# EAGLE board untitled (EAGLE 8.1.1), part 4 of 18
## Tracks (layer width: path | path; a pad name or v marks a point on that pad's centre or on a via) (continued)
S$3328 (continued)
  Bottom 0: 233.07,164.65 233.19,164.95
S$3329
  Bottom 0: 233.19,164.95 233.24,165.27
S$3330
  Bottom 0: 233.24,165.27 233.19,165.59
S$3331
  Bottom 0: 233.19,165.59 233.07,165.89
S$3332
  Bottom 0: 233.07,165.89 232.86,166.14
S$3333
  Bottom 0: 232.86,166.14 232.6,166.33
S$3334
  Bottom 0: 232.6,166.33 232.29,166.44
S$3335
  Bottom 0: 232.29,166.44 232.18,166.44
S$3336
  Bottom 0: 232.18,166.44 232.18,167.7
S$3337
  Bottom 0: 232.18,167.7 232.41,167.45
S$3338
  Bottom 0: 232.41,167.45 232.71,167.26
S$3339
  Bottom 0: 232.71,167.26 233.03,167.16
S$3340
  Bottom 0: 233.03,167.16 233.38,167.14
S$3341
  Bottom 0: 233.38,167.14 233.73,167.2
S$3342
  Bottom 0: 233.73,167.2 234.05,167.35
S$3343
  Bottom 0: 234.05,167.35 234.31,167.57
S$3344
  Bottom 0: 234.31,167.57 234.52,167.86
S$3345
  Bottom 0: 234.52,167.86 234.65,168.18
S$3346
  Bottom 0: 234.65,168.18 234.7,168.53
S$3347
  Bottom 0: 234.7,168.53 234.65,168.87
S$3348
  Bottom 0: 234.65,168.87 234.52,169.2
S$3349
  Bottom 0: 234.52,169.2 234.31,169.48
S$3350
  Bottom 0: 234.31,169.48 234.05,169.71
S$3351
  Bottom 0: 234.05,169.71 233.73,169.86
S$3352
  Bottom 0: 233.73,169.86 233.38,169.92
S$3353
  Bottom 0: 233.38,169.92 233.03,169.9
S$3354
  Bottom 0: 233.03,169.9 232.71,169.79
S$3355
  Bottom 0: 232.71,169.79 232.41,169.61
S$3356
  Bottom 0: 232.41,169.61 232.18,169.36
S$3357
  Bottom 0: 232.18,169.36 232.18,174.4
S$3358
  Bottom 0: 232.18,174.4 234.88,177.1
S$3359
  Bottom 0: 234.88,177.1 234.93,177.17
S$3360
  Bottom 0: 234.93,177.17 234.95,177.2
S$3361
  Bottom 0: 234.95,177.2 234.96,177.24
S$3362
  Bottom 0: 234.96,177.24 235,177.3
S$3363
  Bottom 0: 235,177.3 235,177.36
S$3364
  Bottom 0: 235,177.36 235.01,177.42
S$3365
  Bottom 0: 235.01,177.42 235.01,177.55
S$3366
  Bottom 0: 235.01,177.55 235.46,177.55
S$3367
  Bottom 0: 235.46,177.55 235.53,177.56
S$3368
  Bottom 0: 235.53,177.56 235.6,177.6
S$3369
  Bottom 0: 235.6,177.6 235.66,177.65
S$3370
  Bottom 0: 235.66,177.65 235.7,177.72
S$3371
  Bottom 0: 235.7,177.72 235.71,177.8
S$3372
  Bottom 0: 235.71,177.8 235.71,179.58
S$3373
  Bottom 0: 235.71,179.58 235.7,179.65
S$3374
  Bottom 0: 235.7,179.65 235.66,179.72
S$3375
  Bottom 0: 235.66,179.72 235.6,179.78
S$3376
  Bottom 0: 235.6,179.78 235.53,179.82
S$3377
  Bottom 0: 235.53,179.82 235.46,179.83
S$3378
  Bottom 0: 235.46,179.83 233.68,179.83
S$3379
  Bottom 0: 233.68,179.83 233.6,179.82
S$3380
  Bottom 0: 233.6,179.82 233.53,179.78
S$3381
  Bottom 0: 233.53,179.78 233.48,179.72
S$3382
  Bottom 0: 233.48,179.72 233.44,179.65
S$3383
  Bottom 0: 233.44,179.65 233.43,179.58
S$3384
  Bottom 0: 233.43,179.58 233.43,177.8
S$3385
  Bottom 0: 233.43,177.8 233.44,177.72
S$3386
  Bottom 0: 233.44,177.72 233.48,177.65
S$3387
  Bottom 0: 233.48,177.65 233.53,177.6
S$3388
  Bottom 0: 233.53,177.6 233.6,177.56
S$3389
  Bottom 0: 233.6,177.56 233.68,177.55
S$3390
  Bottom 0: 233.68,177.55 234.07,177.55
S$3391
  Bottom 0: 234.07,177.55 231.42,174.9
S$3392
  Bottom 0: 231.42,174.9 231.38,174.84
S$3393
  Bottom 0: 231.38,174.84 231.34,174.78
S$3394
  Bottom 0: 231.34,174.78 231.31,174.72
S$3395
  Bottom 0: 231.31,174.72 231.29,174.66
S$3396
  Bottom 0: 231.29,174.66 231.29,174.58
S$3397
  Bottom 0: 231.29,174.58 231.29,166.18
S$3398
  Bottom 0: 231.29,166.18 231.12,166.02
S$3399
  Bottom 0: 231.12,166.02 230.95,165.75
S$3400
  Bottom 0: 230.95,165.75 230.87,165.43
S$3401
  Bottom 0: 230.87,165.43 230.87,165.1
S$3402
  Bottom 0: 230.87,165.1 230.95,164.79
S$3403
  Bottom 0: 230.95,164.79 231.12,164.52
S$3404
  Bottom 0: 231.12,164.52 231.36,164.29
S$3405
  Bottom 0: 231.36,164.29 231.65,164.15
S$3406
  Bottom 0: 231.65,164.15 231.97,164.08
S$3407
  Bottom 0: 239.59,164.08 239.92,164.1
S$3408
  Bottom 0: 239.92,164.1 240.22,164.21
S$3409
  Bottom 0: 240.22,164.21 240.49,164.39
S$3410
  Bottom 0: 240.49,164.39 240.69,164.65
S$3411
  Bottom 0: 240.69,164.65 240.82,164.95
S$3412
  Bottom 0: 240.82,164.95 240.87,165.27
S$3413
  Bottom 0: 240.87,165.27 240.82,165.59
S$3414
  Bottom 0: 240.82,165.59 240.69,165.89
S$3415
  Bottom 0: 240.69,165.89 240.49,166.14
S$3416
  Bottom 0: 240.49,166.14 240.22,166.33
S$3417
  Bottom 0: 240.22,166.33 239.92,166.44
S$3418
  Bottom 0: 239.92,166.44 239.59,166.46
S$3419
  Bottom 0: 239.59,166.46 239.27,166.39
S$3420
  Bottom 0: 239.27,166.39 238.98,166.24
S$3421
  Bottom 0: 238.98,166.24 238.75,166.02
S$3422
  Bottom 0: 238.75,166.02 238.58,165.75
S$3423
  Bottom 0: 238.58,165.75 238.49,165.43
S$3424
  Bottom 0: 238.49,165.43 238.49,165.1
S$3425
  Bottom 0: 238.49,165.1 238.58,164.79
S$3426
  Bottom 0: 238.58,164.79 238.75,164.52
S$3427
  Bottom 0: 238.75,164.52 238.98,164.29
S$3428
  Bottom 0: 238.98,164.29 239.27,164.15
S$3429
  Bottom 0: 239.27,164.15 239.59,164.08
S$3430
  Bottom 0: 41.45,164.08 41.78,164.1
S$3431
  Bottom 0: 41.78,164.1 42.08,164.21
S$3432
  Bottom 0: 42.08,164.21 42.35,164.39
S$3433
  Bottom 0: 42.35,164.39 42.55,164.65
S$3434
  Bottom 0: 42.55,164.65 42.68,164.95
S$3435
  Bottom 0: 42.68,164.95 42.73,165.27
S$3436
  Bottom 0: 42.73,165.27 42.68,165.59
S$3437
  Bottom 0: 42.68,165.59 42.55,165.89
S$3438
  Bottom 0: 42.55,165.89 42.35,166.14
S$3439
  Bottom 0: 42.35,166.14 42.08,166.33
S$3440
  Bottom 0: 42.08,166.33 41.78,166.44
S$3441
  Bottom 0: 41.78,166.44 41.66,166.44
S$3442
  Bottom 0: 41.66,166.44 41.66,167.73
S$3443
  Bottom 0: 41.66,167.73 41.67,167.71
S$3444
  Bottom 0: 41.67,167.71 41.91,167.45
S$3445
  Bottom 0: 41.91,167.45 42.2,167.26
S$3446
  Bottom 0: 42.2,167.26 42.53,167.16
S$3447
  Bottom 0: 42.53,167.16 42.88,167.14
S$3448
  Bottom 0: 42.88,167.14 43.23,167.2
S$3449
  Bottom 0: 43.23,167.2 43.55,167.35
S$3450
  Bottom 0: 43.55,167.35 43.81,167.57
S$3451
  Bottom 0: 43.81,167.57 44.02,167.86
S$3452
  Bottom 0: 44.02,167.86 44.15,168.18
S$3453
  Bottom 0: 44.15,168.18 44.2,168.53
S$3454
  Bottom 0: 44.2,168.53 44.15,168.87
S$3455
  Bottom 0: 44.15,168.87 44.02,169.2
S$3456
  Bottom 0: 44.02,169.2 43.81,169.48
S$3457
  Bottom 0: 43.81,169.48 43.55,169.71
S$3458
  Bottom 0: 43.55,169.71 43.23,169.86
S$3459
  Bottom 0: 43.23,169.86 42.88,169.92
S$3460
  Bottom 0: 42.88,169.92 42.53,169.9
S$3461
  Bottom 0: 42.53,169.9 42.2,169.79
S$3462
  Bottom 0: 42.2,169.79 41.91,169.61
S$3463
  Bottom 0: 41.91,169.61 41.67,169.35
S$3464
  Bottom 0: 41.67,169.35 41.66,169.34
S$3465
  Bottom 0: 41.66,169.34 41.66,174.39
S$3466
  Bottom 0: 41.66,174.39 44.38,177.1
S$3467
  Bottom 0: 44.38,177.1 44.41,177.16
S$3468
  Bottom 0: 44.41,177.16 44.45,177.2
S$3469
  Bottom 0: 44.45,177.2 44.46,177.25
S$3470
  Bottom 0: 44.46,177.25 44.49,177.3
S$3471
  Bottom 0: 44.49,177.3 44.49,177.36
S$3472
  Bottom 0: 44.49,177.36 44.51,177.42
S$3473
  Bottom 0: 44.51,177.42 44.51,177.55
S$3474
  Bottom 0: 44.51,177.55 44.96,177.55
S$3475
  Bottom 0: 44.96,177.55 45.03,177.56
S$3476
  Bottom 0: 45.03,177.56 45.1,177.6
S$3477
  Bottom 0: 45.1,177.6 45.16,177.65
S$3478
  Bottom 0: 45.16,177.65 45.2,177.72
S$3479
  Bottom 0: 45.2,177.72 45.21,177.8
S$3480
  Bottom 0: 45.21,177.8 45.21,179.58
S$3481
  Bottom 0: 45.21,179.58 45.2,179.65
S$3482
  Bottom 0: 45.2,179.65 45.16,179.72
S$3483
  Bottom 0: 45.16,179.72 45.1,179.78
S$3484
  Bottom 0: 45.1,179.78 45.03,179.82
S$3485
  Bottom 0: 45.03,179.82 44.96,179.83
S$3486
  Bottom 0: 44.96,179.83 43.18,179.83
S$3487
  Bottom 0: 43.18,179.83 43.1,179.82
S$3488
  Bottom 0: 43.1,179.82 43.03,179.78
S$3489
  Bottom 0: 43.03,179.78 42.98,179.72
S$3490
  Bottom 0: 42.98,179.72 42.93,179.65
S$3491
  Bottom 0: 42.93,179.65 42.93,179.58
S$3492
  Bottom 0: 42.93,179.58 42.93,177.8
S$3493
  Bottom 0: 42.93,177.8 42.93,177.72
S$3494
  Bottom 0: 42.93,177.72 42.98,177.65
S$3495
  Bottom 0: 42.98,177.65 43.03,177.6
S$3496
  Bottom 0: 43.03,177.6 43.1,177.56
S$3497
  Bottom 0: 43.1,177.56 43.18,177.55
S$3498
  Bottom 0: 43.18,177.55 43.57,177.55
S$3499
  Bottom 0: 43.57,177.55 40.91,174.89
S$3500
  Bottom 0: 40.91,174.89 40.86,174.83
S$3501
  Bottom 0: 40.86,174.83 40.83,174.78
S$3502
  Bottom 0: 40.83,174.78 40.8,174.71
S$3503
  Bottom 0: 40.8,174.71 40.78,174.65
S$3504
  Bottom 0: 40.78,174.65 40.77,174.57
S$3505
  Bottom 0: 40.77,174.57 40.77,166.18
S$3506
  Bottom 0: 40.77,166.18 40.61,166.02
S$3507
  Bottom 0: 40.61,166.02 40.44,165.75
S$3508
  Bottom 0: 40.44,165.75 40.35,165.43
S$3509
  Bottom 0: 40.35,165.43 40.35,165.1
S$3510
  Bottom 0: 40.35,165.1 40.44,164.79
S$3511
  Bottom 0: 40.44,164.79 40.61,164.52
S$3512
  Bottom 0: 40.61,164.52 40.84,164.29
S$3513
  Bottom 0: 40.84,164.29 41.13,164.15
S$3514
  Bottom 0: 41.13,164.15 41.45,164.08
S$3515
  Bottom 0: 3.35,164.08 3.67,164.1
S$3516
  Bottom 0: 3.67,164.1 3.98,164.21
S$3517
  Bottom 0: 3.98,164.21 4.24,164.39
S$3518
  Bottom 0: 4.24,164.39 4.45,164.65
S$3519
  Bottom 0: 4.45,164.65 4.58,164.95
S$3520
  Bottom 0: 4.58,164.95 4.62,165.27
S$3521
  Bottom 0: 4.62,165.27 4.58,165.59
S$3522
  Bottom 0: 4.58,165.59 4.45,165.89
S$3523
  Bottom 0: 4.45,165.89 4.24,166.14
S$3524
  Bottom 0: 4.24,166.14 3.98,166.33
S$3525
  Bottom 0: 3.98,166.33 3.67,166.44
S$3526
  Bottom 0: 3.67,166.44 3.56,166.44
S$3527
  Bottom 0: 3.56,166.44 3.56,167.73
S$3528
  Bottom 0: 3.56,167.73 3.57,167.71
S$3529
  Bottom 0: 3.57,167.71 3.81,167.45
S$3530
  Bottom 0: 3.81,167.45 4.11,167.26
S$3531
  Bottom 0: 4.11,167.26 4.43,167.16
S$3532
  Bottom 0: 4.43,167.16 4.78,167.14
S$3533
  Bottom 0: 4.78,167.14 5.13,167.2
S$3534
  Bottom 0: 5.13,167.2 5.45,167.35
S$3535
  Bottom 0: 5.45,167.35 5.71,167.57
S$3536
  Bottom 0: 5.71,167.57 5.92,167.86
S$3537
  Bottom 0: 5.92,167.86 6.05,168.18
S$3538
  Bottom 0: 6.05,168.18 6.1,168.53
S$3539
  Bottom 0: 6.1,168.53 6.05,168.87
S$3540
  Bottom 0: 6.05,168.87 5.92,169.2
S$3541
  Bottom 0: 5.92,169.2 5.71,169.48
S$3542
  Bottom 0: 5.71,169.48 5.45,169.71
S$3543
  Bottom 0: 5.45,169.71 5.13,169.86
S$3544
  Bottom 0: 5.13,169.86 4.78,169.92
S$3545
  Bottom 0: 4.78,169.92 4.43,169.9
S$3546
  Bottom 0: 4.43,169.9 4.11,169.79
S$3547
  Bottom 0: 4.11,169.79 3.81,169.61
S$3548
  Bottom 0: 3.81,169.61 3.57,169.35
S$3549
  Bottom 0: 3.57,169.35 3.56,169.34
S$3550
  Bottom 0: 3.56,169.34 3.56,174.38
S$3551
  Bottom 0: 3.56,174.38 6.28,177.1
S$3552
  Bottom 0: 6.28,177.1 6.32,177.17
S$3553
  Bottom 0: 6.32,177.17 6.35,177.2
S$3554
  Bottom 0: 6.35,177.2 6.36,177.24
S$3555
  Bottom 0: 6.36,177.24 6.4,177.3
S$3556
  Bottom 0: 6.4,177.3 6.4,177.36
S$3557
  Bottom 0: 6.4,177.36 6.41,177.42
S$3558
  Bottom 0: 6.41,177.42 6.41,177.55
S$3559
  Bottom 0: 6.41,177.55 6.86,177.55
S$3560
  Bottom 0: 6.86,177.55 6.93,177.56
S$3561
  Bottom 0: 6.93,177.56 7,177.6
S$3562
  Bottom 0: 7,177.6 7.06,177.65
S$3563
  Bottom 0: 7.06,177.65 7.1,177.72
S$3564
  Bottom 0: 7.1,177.72 7.11,177.8
S$3565
  Bottom 0: 7.11,177.8 7.11,179.58
S$3566
  Bottom 0: 7.11,179.58 7.1,179.65
S$3567
  Bottom 0: 7.1,179.65 7.06,179.72
S$3568
  Bottom 0: 7.06,179.72 7,179.78
S$3569
  Bottom 0: 7,179.78 6.93,179.82
S$3570
  Bottom 0: 6.93,179.82 6.86,179.83
S$3571
  Bottom 0: 6.86,179.83 5.08,179.83
S$3572
  Bottom 0: 5.08,179.83 5,179.82
S$3573
  Bottom 0: 5,179.82 4.93,179.78
S$3574
  Bottom 0: 4.93,179.78 4.87,179.72
S$3575
  Bottom 0: 4.87,179.72 4.84,179.65
S$3576
  Bottom 0: 4.84,179.65 4.83,179.58
S$3577
  Bottom 0: 4.83,179.58 4.83,177.8
S$3578
  Bottom 0: 4.83,177.8 4.84,177.72
S$3579
  Bottom 0: 4.84,177.72 4.87,177.65
S$3580
  Bottom 0: 4.87,177.65 4.93,177.6
S$3581
  Bottom 0: 4.93,177.6 5,177.56
S$3582
  Bottom 0: 5,177.56 5.08,177.55
S$3583
  Bottom 0: 5.08,177.55 5.46,177.55
S$3584
  Bottom 0: 5.46,177.55 2.8,174.88
S$3585
  Bottom 0: 2.8,174.88 2.76,174.83
S$3586
  Bottom 0: 2.76,174.83 2.72,174.77
S$3587
  Bottom 0: 2.72,174.77 2.7,174.71
S$3588
  Bottom 0: 2.7,174.71 2.68,174.64
S$3589
  Bottom 0: 2.68,174.64 2.68,174.57
S$3590
  Bottom 0: 2.68,174.57 2.68,166.19
S$3591
  Bottom 0: 2.68,166.19 2.5,166.02
S$3592
  Bottom 0: 2.5,166.02 2.33,165.75
S$3593
  Bottom 0: 2.33,165.75 2.24,165.43
S$3594
  Bottom 0: 2.24,165.43 2.24,165.1
S$3595
  Bottom 0: 2.24,165.1 2.33,164.79
S$3596
  Bottom 0: 2.33,164.79 2.5,164.52
S$3597
  Bottom 0: 2.5,164.52 2.74,164.29
S$3598
  Bottom 0: 2.74,164.29 3.03,164.15
S$3599
  Bottom 0: 3.03,164.15 3.35,164.08
S$3600
  Bottom 0: 60.5,164.08 60.83,164.1
S$3601
  Bottom 0: 60.83,164.1 61.13,164.21
S$3602
  Bottom 0: 61.13,164.21 61.4,164.4
S$3603
  Bottom 0: 61.4,164.4 61.6,164.65
S$3604
  Bottom 0: 61.6,164.65 61.73,164.95
S$3605
  Bottom 0: 61.73,164.95 61.78,165.27
S$3606
  Bottom 0: 61.78,165.27 61.73,165.59
S$3607
  Bottom 0: 61.73,165.59 61.6,165.89
S$3608
  Bottom 0: 61.6,165.89 61.4,166.15
S$3609
  Bottom 0: 61.4,166.15 61.13,166.33
S$3610
  Bottom 0: 61.13,166.33 60.83,166.44
S$3611
  Bottom 0: 60.83,166.44 60.71,166.44
S$3612
  Bottom 0: 60.71,166.44 60.71,167.72
S$3613
  Bottom 0: 60.71,167.72 60.72,167.71
S$3614
  Bottom 0: 60.72,167.71 60.96,167.45
S$3615
  Bottom 0: 60.96,167.45 61.25,167.26
S$3616
  Bottom 0: 61.25,167.26 61.59,167.16
S$3617
  Bottom 0: 61.59,167.16 61.94,167.14
S$3618
  Bottom 0: 61.94,167.14 62.28,167.2
S$3619
  Bottom 0: 62.28,167.2 62.6,167.35
S$3620
  Bottom 0: 62.6,167.35 62.87,167.57
S$3621
  Bottom 0: 62.87,167.57 63.07,167.86
S$3622
  Bottom 0: 63.07,167.86 63.2,168.18
S$3623
  Bottom 0: 63.2,168.18 63.25,168.53
S$3624
  Bottom 0: 63.25,168.53 63.2,168.87
S$3625
  Bottom 0: 63.2,168.87 63.07,169.2
S$3626
  Bottom 0: 63.07,169.2 62.87,169.48
S$3627
  Bottom 0: 62.87,169.48 62.6,169.71
S$3628
  Bottom 0: 62.6,169.71 62.28,169.86
S$3629
  Bottom 0: 62.28,169.86 61.94,169.92
S$3630
  Bottom 0: 61.94,169.92 61.59,169.9
S$3631
  Bottom 0: 61.59,169.9 61.25,169.79
S$3632
  Bottom 0: 61.25,169.79 60.96,169.61
S$3633
  Bottom 0: 60.96,169.61 60.72,169.35
S$3634
  Bottom 0: 60.72,169.35 60.71,169.35
S$3635
  Bottom 0: 60.71,169.35 60.71,174.4
S$3636
  Bottom 0: 60.71,174.4 63.43,177.1
S$3637
  Bottom 0: 63.43,177.1 63.46,177.16
S$3638
  Bottom 0: 63.46,177.16 63.5,177.2
S$3639
  Bottom 0: 63.5,177.2 63.51,177.25
S$3640
  Bottom 0: 63.51,177.25 63.54,177.3
S$3641
  Bottom 0: 63.54,177.3 63.54,177.36
S$3642
  Bottom 0: 63.54,177.36 63.56,177.42
S$3643
  Bottom 0: 63.56,177.42 63.56,177.55
S$3644
  Bottom 0: 63.56,177.55 64.01,177.55
S$3645
  Bottom 0: 64.01,177.55 64.08,177.56
S$3646
  Bottom 0: 64.08,177.56 64.16,177.6
S$3647
  Bottom 0: 64.16,177.6 64.21,177.65
S$3648
  Bottom 0: 64.21,177.65 64.25,177.72
S$3649
  Bottom 0: 64.25,177.72 64.26,177.8
S$3650
  Bottom 0: 64.26,177.8 64.26,179.58
S$3651
  Bottom 0: 64.26,179.58 64.25,179.65
S$3652
  Bottom 0: 64.25,179.65 64.21,179.72
S$3653
  Bottom 0: 64.21,179.72 64.16,179.78
S$3654
  Bottom 0: 64.16,179.78 64.08,179.82
S$3655
  Bottom 0: 64.08,179.82 64.01,179.83
S$3656
  Bottom 0: 64.01,179.83 62.23,179.83
S$3657
  Bottom 0: 62.23,179.83 62.15,179.82
S$3658
  Bottom 0: 62.15,179.82 62.08,179.78
S$3659
  Bottom 0: 62.08,179.78 62.03,179.72
S$3660
  Bottom 0: 62.03,179.72 61.98,179.65
S$3661
  Bottom 0: 61.98,179.65 61.98,179.58
S$3662
  Bottom 0: 61.98,179.58 61.98,177.8
S$3663
  Bottom 0: 61.98,177.8 61.98,177.72
S$3664
  Bottom 0: 61.98,177.72 62.03,177.65
S$3665
  Bottom 0: 62.03,177.65 62.08,177.6
S$3666
  Bottom 0: 62.08,177.6 62.15,177.56
S$3667
  Bottom 0: 62.15,177.56 62.23,177.55
S$3668
  Bottom 0: 62.23,177.55 62.62,177.55
S$3669
  Bottom 0: 62.62,177.55 59.96,174.89
S$3670
  Bottom 0: 59.96,174.89 59.92,174.84
S$3671
  Bottom 0: 59.92,174.84 59.88,174.78
S$3672
  Bottom 0: 59.88,174.78 59.85,174.72
S$3673
  Bottom 0: 59.85,174.72 59.84,174.65
S$3674
  Bottom 0: 59.84,174.65 59.83,174.58
S$3675
  Bottom 0: 59.83,174.58 59.83,166.19
S$3676
  Bottom 0: 59.83,166.19 59.66,166.03
S$3677
  Bottom 0: 59.66,166.03 59.49,165.75
S$3678
  Bottom 0: 59.49,165.75 59.4,165.43
S$3679
  Bottom 0: 59.4,165.43 59.4,165.11
S$3680
  Bottom 0: 59.4,165.11 59.49,164.79
S$3681
  Bottom 0: 59.49,164.79 59.66,164.52
S$3682
  Bottom 0: 59.66,164.52 59.89,164.3
S$3683
  Bottom 0: 59.89,164.3 60.18,164.15
S$3684
  Bottom 0: 60.18,164.15 60.5,164.08
S$3685
  Bottom 0: 16.5,168.1 17.02,168.1
S$3686
  Bottom 0: 17.02,168.1 17.53,168.19
S$3687
  Bottom 0: 17.53,168.19 18.02,168.36
S$3688
  Bottom 0: 18.02,168.36 18.48,168.6
S$3689
  Bottom 0: 18.48,168.6 18.89,168.92
S$3690
  Bottom 0: 18.89,168.92 19.24,169.3
S$3691
  Bottom 0: 19.24,169.3 19.52,169.73
S$3692
  Bottom 0: 19.52,169.73 19.73,170.21
S$3693
  Bottom 0: 19.73,170.21 19.86,170.71
S$3694
  Bottom 0: 19.86,170.71 19.9,171.23
S$3695
  Bottom 0: 19.9,171.23 19.86,171.75
S$3696
  Bottom 0: 19.86,171.75 19.73,172.24
S$3697
  Bottom 0: 19.73,172.24 19.52,172.72
S$3698
  Bottom 0: 19.52,172.72 19.24,173.15
S$3699
  Bottom 0: 19.24,173.15 18.89,173.53
S$3700
  Bottom 0: 18.89,173.53 18.48,173.85
S$3701
  Bottom 0: 18.48,173.85 18.02,174.1
S$3702
  Bottom 0: 18.02,174.1 17.53,174.26
S$3703
  Bottom 0: 17.53,174.26 17.02,174.35
S$3704
  Bottom 0: 17.02,174.35 16.5,174.35
S$3705
  Bottom 0: 16.5,174.35 16,174.26
S$3706
  Bottom 0: 16,174.26 15.5,174.1
S$3707
  Bottom 0: 15.5,174.1 15.05,173.85
S$3708
  Bottom 0: 15.05,173.85 14.64,173.53
S$3709
  Bottom 0: 14.64,173.53 14.29,173.15
S$3710
  Bottom 0: 14.29,173.15 14,172.72
S$3711
  Bottom 0: 14,172.72 13.79,172.24
S$3712
  Bottom 0: 13.79,172.24 13.67,171.75
S$3713
  Bottom 0: 13.67,171.75 13.63,171.23
S$3714
  Bottom 0: 13.63,171.23 13.67,170.71
S$3715
  Bottom 0: 13.67,170.71 13.79,170.21
S$3716
  Bottom 0: 13.79,170.21 14,169.73
S$3717
  Bottom 0: 14,169.73 14.29,169.3
S$3718
  Bottom 0: 14.29,169.3 14.64,168.92
S$3719
  Bottom 0: 14.64,168.92 15.05,168.6
S$3720
  Bottom 0: 15.05,168.6 15.5,168.36
S$3721
  Bottom 0: 15.5,168.36 16,168.19
S$3722
  Bottom 0: 16,168.19 16.5,168.1
S$3723
  Bottom 0: 54.95,169.02 55.24,169.09
S$3724
  Bottom 0: 55.24,169.09 55.5,169.24
S$3725
  Bottom 0: 55.5,169.24 55.71,169.46
S$3726
  Bottom 0: 55.71,169.46 55.84,169.73
S$3727
  Bottom 0: 55.84,169.73 55.88,170.03
S$3728
  Bottom 0: 55.88,170.03 55.84,170.33
S$3729
  Bottom 0: 55.84,170.33 55.71,170.61
S$3730
  Bottom 0: 55.71,170.61 55.5,170.82
S$3731
  Bottom 0: 55.5,170.82 55.24,170.98
S$3732
  Bottom 0: 55.24,170.98 54.95,171.04
S$3733
  Bottom 0: 54.95,171.04 54.64,171.02
S$3734
  Bottom 0: 54.64,171.02 54.36,170.91
S$3735
  Bottom 0: 54.36,170.91 54.12,170.72
S$3736
  Bottom 0: 54.12,170.72 53.95,170.47
S$3737
  Bottom 0: 53.95,170.47 53.86,170.19
S$3738
  Bottom 0: 53.86,170.19 53.86,169.88
S$3739
  Bottom 0: 53.86,169.88 53.95,169.59
S$3740
  Bottom 0: 53.95,169.59 54.12,169.34
S$3741
  Bottom 0: 54.12,169.34 54.36,169.15
S$3742
  Bottom 0: 54.36,169.15 54.64,169.04
S$3743
  Bottom 0: 54.64,169.04 54.95,169.02
S$3744
  Bottom 0: 207.36,169.03 207.66,169.09
S$3745
  Bottom 0: 207.66,169.09 207.92,169.25
S$3746
  Bottom 0: 207.92,169.25 208.12,169.46
S$3747
  Bottom 0: 208.12,169.46 208.25,169.74
S$3748
  Bottom 0: 208.25,169.74 208.3,170.04
S$3749
  Bottom 0: 208.3,170.04 208.25,170.34
S$3750
  Bottom 0: 208.25,170.34 208.12,170.61
S$3751
  Bottom 0: 208.12,170.61 207.92,170.83
S$3752
  Bottom 0: 207.92,170.83 207.66,170.98
S$3753
  Bottom 0: 207.66,170.98 207.36,171.05
S$3754
  Bottom 0: 207.36,171.05 207.06,171.03
S$3755
  Bottom 0: 207.06,171.03 206.78,170.92
S$3756
  Bottom 0: 206.78,170.92 206.54,170.73
S$3757
  Bottom 0: 206.54,170.73 206.37,170.48
S$3758
  Bottom 0: 206.37,170.48 206.28,170.19
S$3759
  Bottom 0: 206.28,170.19 206.28,169.88
S$3760
  Bottom 0: 206.28,169.88 206.37,169.6
S$3761
  Bottom 0: 206.37,169.6 206.54,169.35
S$3762
  Bottom 0: 206.54,169.35 206.78,169.16
S$3763
  Bottom 0: 206.78,169.16 207.06,169.05
S$3764
  Bottom 0: 207.06,169.05 207.36,169.03
S$3765
  Bottom 0: 68.28,169.68 68.63,169.74
S$3766
  Bottom 0: 68.63,169.74 68.95,169.89
S$3767
  Bottom 0: 68.95,169.89 69.22,170.11
S$3768
  Bottom 0: 69.22,170.11 69.42,170.4
S$3769
  Bottom 0: 69.42,170.4 69.55,170.72
S$3770
  Bottom 0: 69.55,170.72 69.6,171.07
S$3771
  Bottom 0: 69.6,171.07 69.55,171.41
S$3772
  Bottom 0: 69.55,171.41 69.42,171.74
S$3773
  Bottom 0: 69.42,171.74 69.22,172.02
S$3774
  Bottom 0: 69.22,172.02 68.95,172.25
S$3775
  Bottom 0: 68.95,172.25 68.63,172.4
S$3776
  Bottom 0: 68.63,172.4 68.28,172.46
S$3777
  Bottom 0: 68.28,172.46 67.94,172.44
S$3778
  Bottom 0: 67.94,172.44 67.6,172.33
S$3779
  Bottom 0: 67.6,172.33 67.31,172.15
S$3780
  Bottom 0: 67.31,172.15 67.07,171.89
S$3781
  Bottom 0: 67.07,171.89 66.9,171.58
S$3782
  Bottom 0: 66.9,171.58 66.81,171.24
S$3783
  Bottom 0: 66.81,171.24 66.81,170.9
S$3784
  Bottom 0: 66.81,170.9 66.9,170.56
S$3785
  Bottom 0: 66.9,170.56 67.07,170.25
S$3786
  Bottom 0: 67.07,170.25 67.31,169.99
S$3787
  Bottom 0: 67.31,169.99 67.6,169.8
S$3788
  Bottom 0: 67.6,169.8 67.94,169.7
S$3789
  Bottom 0: 67.94,169.7 68.28,169.68
S$3790
  Bottom 0: 49.23,169.68 49.58,169.74
S$3791
  Bottom 0: 49.58,169.74 49.9,169.89
S$3792
  Bottom 0: 49.9,169.89 50.16,170.11
S$3793
  Bottom 0: 50.16,170.11 50.37,170.4
S$3794
  Bottom 0: 50.37,170.4 50.5,170.72
S$3795
  Bottom 0: 50.5,170.72 50.55,171.07
S$3796
  Bottom 0: 50.55,171.07 50.5,171.41
S$3797
  Bottom 0: 50.5,171.41 50.37,171.74
S$3798
  Bottom 0: 50.37,171.74 50.16,172.02
S$3799
  Bottom 0: 50.16,172.02 49.9,172.25
S$3800
  Bottom 0: 49.9,172.25 49.58,172.4
S$3801
  Bottom 0: 49.58,172.4 49.23,172.46
S$3802
  Bottom 0: 49.23,172.46 48.88,172.44
S$3803
  Bottom 0: 48.88,172.44 48.55,172.33
S$3804
  Bottom 0: 48.55,172.33 48.26,172.15
S$3805
  Bottom 0: 48.26,172.15 48.02,171.89
S$3806
  Bottom 0: 48.02,171.89 47.85,171.58
S$3807
  Bottom 0: 47.85,171.58 47.76,171.24
S$3808
  Bottom 0: 47.76,171.24 47.76,170.9
S$3809
  Bottom 0: 47.76,170.9 47.85,170.56
S$3810
  Bottom 0: 47.85,170.56 48.02,170.25
S$3811
  Bottom 0: 48.02,170.25 48.26,169.99
S$3812
  Bottom 0: 48.26,169.99 48.55,169.8
S$3813
  Bottom 0: 48.55,169.8 48.88,169.7
S$3814
  Bottom 0: 48.88,169.7 49.23,169.68
S$3815
  Bottom 0: 235.84,171.32 236.29,171.37
S$3816
  Bottom 0: 236.29,171.37 236.71,171.5
S$3817
  Bottom 0: 236.71,171.5 237.11,171.71
S$3818
  Bottom 0: 237.11,171.71 237.45,171.99
S$3819
  Bottom 0: 237.45,171.99 237.74,172.34
S$3820
  Bottom 0: 237.74,172.34 237.95,172.74
S$3821
  Bottom 0: 237.95,172.74 238.08,173.16
S$3822
  Bottom 0: 238.08,173.16 238.12,173.61
S$3823
  Bottom 0: 238.12,173.61 238.08,174.06
S$3824
  Bottom 0: 238.08,174.06 237.95,174.48
S$3825
  Bottom 0: 237.95,174.48 237.74,174.88
S$3826
  Bottom 0: 237.74,174.88 237.45,175.22
S$3827
  Bottom 0: 237.45,175.22 237.11,175.51
S$3828
  Bottom 0: 237.11,175.51 236.71,175.72
S$3829
  Bottom 0: 236.71,175.72 236.29,175.85
S$3830
  Bottom 0: 236.29,175.85 235.84,175.9
S$3831
  Bottom 0: 235.84,175.9 235.39,175.85
S$3832
  Bottom 0: 235.39,175.85 234.97,175.72
S$3833
  Bottom 0: 234.97,175.72 234.57,175.51
S$3834
  Bottom 0: 234.57,175.51 234.22,175.22
S$3835
  Bottom 0: 234.22,175.22 233.94,174.88
S$3836
  Bottom 0: 233.94,174.88 233.73,174.48
S$3837
  Bottom 0: 233.73,174.48 233.6,174.06
S$3838
  Bottom 0: 233.6,174.06 233.55,173.61
S$3839
  Bottom 0: 233.55,173.61 233.6,173.16
S$3840
  Bottom 0: 233.6,173.16 233.73,172.74
S$3841
  Bottom 0: 233.73,172.74 233.94,172.34
S$3842
  Bottom 0: 233.94,172.34 234.22,171.99
S$3843
  Bottom 0: 234.22,171.99 234.57,171.71
S$3844
  Bottom 0: 234.57,171.71 234.97,171.5
S$3845
  Bottom 0: 234.97,171.5 235.39,171.37
S$3846
  Bottom 0: 235.39,171.37 235.84,171.32
S$3847
  Bottom 0: 178.69,171.32 179.14,171.37
S$3848
  Bottom 0: 179.14,171.37 179.56,171.5
S$3849
  Bottom 0: 179.56,171.5 179.96,171.71
S$3850
  Bottom 0: 179.96,171.71 180.3,171.99
S$3851
  Bottom 0: 180.3,171.99 180.59,172.34
S$3852
  Bottom 0: 180.59,172.34 180.8,172.74
S$3853
  Bottom 0: 180.8,172.74 180.93,173.16
S$3854
  Bottom 0: 180.93,173.16 180.97,173.61
S$3855
  Bottom 0: 180.97,173.61 180.93,174.06
S$3856
  Bottom 0: 180.93,174.06 180.8,174.48
S$3857
  Bottom 0: 180.8,174.48 180.59,174.88
S$3858
  Bottom 0: 180.59,174.88 180.3,175.22
S$3859
  Bottom 0: 180.3,175.22 179.96,175.51
S$3860
  Bottom 0: 179.96,175.51 179.56,175.72
S$3861
  Bottom 0: 179.56,175.72 179.14,175.85
S$3862
  Bottom 0: 179.14,175.85 178.69,175.9
S$3863
  Bottom 0: 178.69,175.9 178.24,175.85
S$3864
  Bottom 0: 178.24,175.85 177.81,175.72
S$3865
  Bottom 0: 177.81,175.72 177.42,175.51
S$3866
  Bottom 0: 177.42,175.51 177.07,175.22
S$3867
  Bottom 0: 177.07,175.22 176.79,174.88
S$3868
  Bottom 0: 176.79,174.88 176.58,174.48
S$3869
  Bottom 0: 176.58,174.48 176.45,174.06
S$3870
  Bottom 0: 176.45,174.06 176.4,173.61
S$3871
  Bottom 0: 176.4,173.61 176.45,173.16
S$3872
  Bottom 0: 176.45,173.16 176.58,172.74
S$3873
  Bottom 0: 176.58,172.74 176.79,172.34
S$3874
  Bottom 0: 176.79,172.34 177.07,171.99
S$3875
  Bottom 0: 177.07,171.99 177.42,171.71
S$3876
  Bottom 0: 177.42,171.71 177.81,171.5
S$3877
  Bottom 0: 177.81,171.5 178.24,171.37
S$3878
  Bottom 0: 178.24,171.37 178.69,171.32
S$3879
  Bottom 0: 64.39,171.32 64.84,171.37
S$3880
  Bottom 0: 64.84,171.37 65.26,171.5
S$3881
  Bottom 0: 65.26,171.5 65.66,171.71
S$3882
  Bottom 0: 65.66,171.71 66,171.99
S$3883
  Bottom 0: 66,171.99 66.29,172.34
S$3884
  Bottom 0: 66.29,172.34 66.5,172.74
S$3885
  Bottom 0: 66.5,172.74 66.63,173.16
S$3886
  Bottom 0: 66.63,173.16 66.67,173.61
S$3887
  Bottom 0: 66.67,173.61 66.63,174.06
S$3888
  Bottom 0: 66.63,174.06 66.5,174.48
S$3889
  Bottom 0: 66.5,174.48 66.29,174.88
S$3890
  Bottom 0: 66.29,174.88 66,175.22
S$3891
  Bottom 0: 66,175.22 65.66,175.51
S$3892
  Bottom 0: 65.66,175.51 65.26,175.72
S$3893
  Bottom 0: 65.26,175.72 64.84,175.85
S$3894
  Bottom 0: 64.84,175.85 64.39,175.9
S$3895
  Bottom 0: 64.39,175.9 63.94,175.85
S$3896
  Bottom 0: 63.94,175.85 63.51,175.72
S$3897
  Bottom 0: 63.51,175.72 63.12,175.51
S$3898
  Bottom 0: 63.12,175.51 62.77,175.22
S$3899
  Bottom 0: 62.77,175.22 62.49,174.88
S$3900
  Bottom 0: 62.49,174.88 62.27,174.48
S$3901
  Bottom 0: 62.27,174.48 62.15,174.06
S$3902
  Bottom 0: 62.15,174.06 62.1,173.61
S$3903
  Bottom 0: 62.1,173.61 62.15,173.16
S$3904
  Bottom 0: 62.15,173.16 62.27,172.74
S$3905
  Bottom 0: 62.27,172.74 62.49,172.34
S$3906
  Bottom 0: 62.49,172.34 62.77,171.99
S$3907
  Bottom 0: 62.77,171.99 63.12,171.71
S$3908
  Bottom 0: 63.12,171.71 63.51,171.5
S$3909
  Bottom 0: 63.51,171.5 63.94,171.37
S$3910
  Bottom 0: 63.94,171.37 64.39,171.32
S$3911
  Bottom 0: 45.34,171.32 45.79,171.37
S$3912
  Bottom 0: 45.79,171.37 46.21,171.5
S$3913
  Bottom 0: 46.21,171.5 46.61,171.71
S$3914
  Bottom 0: 46.61,171.71 46.95,171.99
S$3915
  Bottom 0: 46.95,171.99 47.24,172.34
S$3916
  Bottom 0: 47.24,172.34 47.45,172.74
S$3917
  Bottom 0: 47.45,172.74 47.58,173.16
S$3918
  Bottom 0: 47.58,173.16 47.62,173.61
S$3919
  Bottom 0: 47.62,173.61 47.58,174.06
S$3920
  Bottom 0: 47.58,174.06 47.45,174.48
S$3921
  Bottom 0: 47.45,174.48 47.24,174.88
S$3922
  Bottom 0: 47.24,174.88 46.95,175.22
S$3923
  Bottom 0: 46.95,175.22 46.61,175.51
S$3924
  Bottom 0: 46.61,175.51 46.21,175.72
S$3925
  Bottom 0: 46.21,175.72 45.79,175.85
S$3926
  Bottom 0: 45.79,175.85 45.34,175.9
S$3927
  Bottom 0: 45.34,175.9 44.89,175.85
S$3928
  Bottom 0: 44.89,175.85 44.46,175.72
S$3929
  Bottom 0: 44.46,175.72 44.07,175.51
S$3930
  Bottom 0: 44.07,175.51 43.72,175.22
S$3931
  Bottom 0: 43.72,175.22 43.44,174.88
S$3932
  Bottom 0: 43.44,174.88 43.22,174.48
S$3933
  Bottom 0: 43.22,174.48 43.1,174.06
S$3934
  Bottom 0: 43.1,174.06 43.05,173.61
S$3935
  Bottom 0: 43.05,173.61 43.1,173.16
S$3936
  Bottom 0: 43.1,173.16 43.22,172.74
S$3937
  Bottom 0: 43.22,172.74 43.44,172.34
S$3938
  Bottom 0: 43.44,172.34 43.72,171.99
S$3939
  Bottom 0: 43.72,171.99 44.07,171.71
S$3940
  Bottom 0: 44.07,171.71 44.46,171.5
S$3941
  Bottom 0: 44.46,171.5 44.89,171.37
S$3942
  Bottom 0: 44.89,171.37 45.34,171.32
S$3943
  Bottom 0: 54.95,176.64 55.24,176.71
S$3944
  Bottom 0: 55.24,176.71 55.5,176.86
S$3945
  Bottom 0: 55.5,176.86 55.71,177.08
S$3946
  Bottom 0: 55.71,177.08 55.84,177.35
S$3947
  Bottom 0: 55.84,177.35 55.88,177.65
S$3948
  Bottom 0: 55.88,177.65 55.84,177.95
S$3949
  Bottom 0: 55.84,177.95 55.71,178.23
S$3950
  Bottom 0: 55.71,178.23 55.5,178.44
S$3951
  Bottom 0: 55.5,178.44 55.24,178.6
S$3952
  Bottom 0: 55.24,178.6 54.95,178.66
S$3953
  Bottom 0: 54.95,178.66 54.64,178.64
S$3954
  Bottom 0: 54.64,178.64 54.36,178.53
S$3955
  Bottom 0: 54.36,178.53 54.12,178.34
S$3956
  Bottom 0: 54.12,178.34 53.95,178.09
S$3957
  Bottom 0: 53.95,178.09 53.86,177.81
S$3958
  Bottom 0: 53.86,177.81 53.86,177.5
S$3959
  Bottom 0: 53.86,177.5 53.95,177.21
S$3960
  Bottom 0: 53.95,177.21 54.12,176.96
S$3961
  Bottom 0: 54.12,176.96 54.36,176.77
S$3962
  Bottom 0: 54.36,176.77 54.64,176.66
S$3963
  Bottom 0: 54.64,176.66 54.95,176.64
S$3964
  Bottom 0: 226.41,176.65 226.71,176.71
S$3965
  Bottom 0: 226.71,176.71 226.97,176.87
S$3966
  Bottom 0: 226.97,176.87 227.17,177.08
S$3967
  Bottom 0: 227.17,177.08 227.31,177.36
S$3968
  Bottom 0: 227.31,177.36 227.35,177.66
S$3969
  Bottom 0: 227.35,177.66 227.31,177.96
S$3970
  Bottom 0: 227.31,177.96 227.17,178.23
S$3971
  Bottom 0: 227.17,178.23 226.97,178.45
S$3972
  Bottom 0: 226.97,178.45 226.71,178.6
S$3973
  Bottom 0: 226.71,178.6 226.41,178.67
S$3974
  Bottom 0: 226.41,178.67 226.11,178.65
S$3975
  Bottom 0: 226.11,178.65 225.83,178.54
S$3976
  Bottom 0: 225.83,178.54 225.59,178.35
S$3977
  Bottom 0: 225.59,178.35 225.42,178.1
S$3978
  Bottom 0: 225.42,178.1 225.33,177.81
S$3979
  Bottom 0: 225.33,177.81 225.33,177.5
S$3980
  Bottom 0: 225.33,177.5 225.42,177.22
S$3981
  Bottom 0: 225.42,177.22 225.59,176.97
S$3982
  Bottom 0: 225.59,176.97 225.83,176.78
S$3983
  Bottom 0: 225.83,176.78 226.11,176.67
S$3984
  Bottom 0: 226.11,176.67 226.41,176.65
S$3985
  Bottom 0: 207.36,176.65 207.66,176.71
S$3986
  Bottom 0: 207.66,176.71 207.92,176.87
S$3987
  Bottom 0: 207.92,176.87 208.12,177.08
S$3988
  Bottom 0: 208.12,177.08 208.25,177.36
S$3989
  Bottom 0: 208.25,177.36 208.3,177.66
S$3990
  Bottom 0: 208.3,177.66 208.25,177.96
S$3991
  Bottom 0: 208.25,177.96 208.12,178.23
S$3992
  Bottom 0: 208.12,178.23 207.92,178.45
S$3993
  Bottom 0: 207.92,178.45 207.66,178.6
S$3994
  Bottom 0: 207.66,178.6 207.36,178.67
S$3995
  Bottom 0: 207.36,178.67 207.06,178.65
S$3996
  Bottom 0: 207.06,178.65 206.78,178.54
S$3997
  Bottom 0: 206.78,178.54 206.54,178.35
S$3998
  Bottom 0: 206.54,178.35 206.37,178.1
S$3999
  Bottom 0: 206.37,178.1 206.28,177.81
S$4000
  Bottom 0: 206.28,177.81 206.28,177.5
S$4001
  Bottom 0: 206.28,177.5 206.37,177.22
S$4002
  Bottom 0: 206.37,177.22 206.54,176.97
S$4003
  Bottom 0: 206.54,176.97 206.78,176.78
S$4004
  Bottom 0: 206.78,176.78 207.06,176.67
S$4005
  Bottom 0: 207.06,176.67 207.36,176.65
S$4006
  Bottom 0: 187.12,176.65 187.41,176.71
S$4007
  Bottom 0: 187.41,176.71 187.68,176.87
S$4008
  Bottom 0: 187.68,176.87 187.88,177.08
S$4009
  Bottom 0: 187.88,177.08 188.02,177.36
S$4010
  Bottom 0: 188.02,177.36 188.06,177.66
S$4011
  Bottom 0: 188.06,177.66 188.02,177.96
S$4012
  Bottom 0: 188.02,177.96 187.88,178.23
S$4013
  Bottom 0: 187.88,178.23 187.68,178.45
S$4014
  Bottom 0: 187.68,178.45 187.41,178.6
S$4015
  Bottom 0: 187.41,178.6 187.12,178.67
S$4016
  Bottom 0: 187.12,178.67 186.82,178.65
S$4017
  Bottom 0: 186.82,178.65 186.54,178.54
S$4018
  Bottom 0: 186.54,178.54 186.3,178.35
S$4019
  Bottom 0: 186.3,178.35 186.13,178.1
S$4020
  Bottom 0: 186.13,178.1 186.04,177.81
S$4021
  Bottom 0: 186.04,177.81 186.04,177.5
S$4022
  Bottom 0: 186.04,177.5 186.13,177.22
S$4023
  Bottom 0: 186.13,177.22 186.3,176.97
S$4024
  Bottom 0: 186.3,176.97 186.54,176.78
S$4025
  Bottom 0: 186.54,176.78 186.82,176.67
S$4026
  Bottom 0: 186.82,176.67 187.12,176.65
S$4027
  Bottom 0: 75.19,176.65 75.48,176.71
S$4028
  Bottom 0: 75.48,176.71 75.75,176.87
S$4029
  Bottom 0: 75.75,176.87 75.95,177.08
S$4030
  Bottom 0: 75.95,177.08 76.08,177.36
S$4031
  Bottom 0: 76.08,177.36 76.13,177.66
S$4032
  Bottom 0: 76.13,177.66 76.08,177.96
S$4033
  Bottom 0: 76.08,177.96 75.95,178.23
S$4034
  Bottom 0: 75.95,178.23 75.75,178.45
S$4035
  Bottom 0: 75.75,178.45 75.48,178.6
S$4036
  Bottom 0: 75.48,178.6 75.19,178.67
S$4037
  Bottom 0: 75.19,178.67 74.88,178.65
S$4038
  Bottom 0: 74.88,178.65 74.61,178.54
S$4039
  Bottom 0: 74.61,178.54 74.36,178.35
S$4040
  Bottom 0: 74.36,178.35 74.2,178.1
S$4041
  Bottom 0: 74.2,178.1 74.11,177.81
S$4042
  Bottom 0: 74.11,177.81 74.11,177.5
S$4043
  Bottom 0: 74.11,177.5 74.2,177.22
S$4044
  Bottom 0: 74.2,177.22 74.36,176.97
S$4045
  Bottom 0: 74.36,176.97 74.61,176.78
S$4046
  Bottom 0: 74.61,176.78 74.88,176.67
S$4047
  Bottom 0: 74.88,176.67 75.19,176.65
S$4048
  Bottom 0: 37.08,176.65 37.38,176.71
S$4049
  Bottom 0: 37.38,176.71 37.64,176.87
S$4050
  Bottom 0: 37.64,176.87 37.85,177.08
S$4051
  Bottom 0: 37.85,177.08 37.98,177.36
S$4052
  Bottom 0: 37.98,177.36 38.02,177.66
S$4053
  Bottom 0: 38.02,177.66 37.98,177.96
S$4054
  Bottom 0: 37.98,177.96 37.85,178.23
S$4055
  Bottom 0: 37.85,178.23 37.64,178.45
S$4056
  Bottom 0: 37.64,178.45 37.38,178.6
S$4057
  Bottom 0: 37.38,178.6 37.08,178.67
S$4058
  Bottom 0: 37.08,178.67 36.78,178.65
S$4059
  Bottom 0: 36.78,178.65 36.5,178.54
S$4060
  Bottom 0: 36.5,178.54 36.26,178.35
S$4061
  Bottom 0: 36.26,178.35 36.09,178.1
S$4062
  Bottom 0: 36.09,178.1 36,177.81
S$4063
  Bottom 0: 36,177.81 36,177.5
S$4064
  Bottom 0: 36,177.5 36.09,177.22
S$4065
  Bottom 0: 36.09,177.22 36.26,176.97
S$4066
  Bottom 0: 36.26,176.97 36.5,176.78
S$4067
  Bottom 0: 36.5,176.78 36.78,176.67
S$4068
  Bottom 0: 36.78,176.67 37.08,176.65
S$4069
  Bottom 0: 34.7,176.65 35,176.71
S$4070
  Bottom 0: 35,176.71 35.26,176.87
S$4071
  Bottom 0: 35.26,176.87 35.47,177.08
S$4072
  Bottom 0: 35.47,177.08 35.6,177.36
S$4073
  Bottom 0: 35.6,177.36 35.65,177.66
S$4074
  Bottom 0: 35.65,177.66 35.6,177.96
S$4075
  Bottom 0: 35.6,177.96 35.47,178.23
S$4076
  Bottom 0: 35.47,178.23 35.26,178.45
S$4077
  Bottom 0: 35.26,178.45 35,178.6
S$4078
  Bottom 0: 35,178.6 34.7,178.67
S$4079
  Bottom 0: 34.7,178.67 34.4,178.65
S$4080
  Bottom 0: 34.4,178.65 34.12,178.54
S$4081
  Bottom 0: 34.12,178.54 33.88,178.35
S$4082
  Bottom 0: 33.88,178.35 33.72,178.1
S$4083
  Bottom 0: 33.72,178.1 33.62,177.81
S$4084
  Bottom 0: 33.62,177.81 33.62,177.5
S$4085
  Bottom 0: 33.62,177.5 33.72,177.22
S$4086
  Bottom 0: 33.72,177.22 33.88,176.97
S$4087
  Bottom 0: 33.88,176.97 34.12,176.78
S$4088
  Bottom 0: 34.12,176.78 34.4,176.67
S$4089
  Bottom 0: 34.4,176.67 34.7,176.65
S$4090
  Bottom 0: 281.67,177.1 281.67,177.81
S$4091
  Bottom 0: 281.67,177.81 280.97,177.81
S$4092
  Bottom 0: 280.97,177.81 281.11,177.56
S$4093
  Bottom 0: 281.11,177.56 281.35,177.3
S$4094
  Bottom 0: 281.35,177.3 281.64,177.11
S$4095
  Bottom 0: 281.64,177.11 281.67,177.1
S$4096
  Bottom 0: 282.82,177.11 283,177.19
S$4097
  Bottom 0: 283,177.19 283.27,177.42
S$4098
  Bottom 0: 283.27,177.42 283.47,177.7
S$4099
  Bottom 0: 283.47,177.7 283.51,177.81
S$4100
  Bottom 0: 283.51,177.81 282.82,177.81
S$4101
  Bottom 0: 282.82,177.81 282.82,177.11
S$4102
  Bottom 0: 65.5,177.56 65.82,177.56
S$4103
  Bottom 0: 65.82,177.56 66.13,177.65
S$4104
  Bottom 0: 66.13,177.65 66.41,177.82
S$4105
  Bottom 0: 66.41,177.82 66.62,178.07
S$4106
  Bottom 0: 66.62,178.07 66.76,178.37
S$4107
  Bottom 0: 66.76,178.37 66.8,178.69
S$4108
  Bottom 0: 66.8,178.69 66.76,179.01
S$4109
  Bottom 0: 66.76,179.01 66.62,179.31
S$4110
  Bottom 0: 66.62,179.31 66.41,179.55
S$4111
  Bottom 0: 66.41,179.55 66.13,179.73
S$4112
  Bottom 0: 66.13,179.73 65.82,179.82
S$4113
  Bottom 0: 65.82,179.82 65.5,179.82
S$4114
  Bottom 0: 65.5,179.82 65.19,179.73
S$4115
  Bottom 0: 65.19,179.73 64.91,179.55
S$4116
  Bottom 0: 64.91,179.55 64.7,179.31
S$4117
  Bottom 0: 64.7,179.31 64.56,179.01
S$4118
  Bottom 0: 64.56,179.01 64.52,178.69
S$4119
  Bottom 0: 64.52,178.69 64.56,178.37
S$4120
  Bottom 0: 64.56,178.37 64.7,178.07
S$4121
  Bottom 0: 64.7,178.07 64.91,177.82
S$4122
  Bottom 0: 64.91,177.82 65.19,177.65
S$4123
  Bottom 0: 65.19,177.65 65.5,177.56
S$4124
  Bottom 0: 46.45,177.56 46.77,177.56
S$4125
  Bottom 0: 46.77,177.56 47.08,177.65
S$4126
  Bottom 0: 47.08,177.65 47.36,177.82
S$4127
  Bottom 0: 47.36,177.82 47.57,178.07
S$4128
  Bottom 0: 47.57,178.07 47.71,178.37
S$4129
  Bottom 0: 47.71,178.37 47.75,178.69
S$4130
  Bottom 0: 47.75,178.69 47.71,179.01
S$4131
  Bottom 0: 47.71,179.01 47.57,179.31
S$4132
  Bottom 0: 47.57,179.31 47.36,179.55
S$4133
  Bottom 0: 47.36,179.55 47.08,179.73
S$4134
  Bottom 0: 47.08,179.73 46.77,179.82
S$4135
  Bottom 0: 46.77,179.82 46.45,179.82
S$4136
  Bottom 0: 46.45,179.82 46.14,179.73
S$4137
  Bottom 0: 46.14,179.73 45.86,179.55
S$4138
  Bottom 0: 45.86,179.55 45.65,179.31
S$4139
  Bottom 0: 45.65,179.31 45.51,179.01
S$4140
  Bottom 0: 45.51,179.01 45.47,178.69
S$4141
  Bottom 0: 45.47,178.69 45.51,178.37
S$4142
  Bottom 0: 45.51,178.37 45.65,178.07
S$4143
  Bottom 0: 45.65,178.07 45.86,177.82
S$4144
  Bottom 0: 45.86,177.82 46.14,177.65
S$4145
  Bottom 0: 46.14,177.65 46.45,177.56
S$4146
  Bottom 0: 27.4,177.56 27.72,177.56
S$4147
  Bottom 0: 27.72,177.56 28.03,177.65
S$4148
  Bottom 0: 28.03,177.65 28.31,177.82
S$4149
  Bottom 0: 28.31,177.82 28.52,178.07
S$4150
  Bottom 0: 28.52,178.07 28.66,178.37
S$4151
  Bottom 0: 28.66,178.37 28.7,178.69
S$4152
  Bottom 0: 28.7,178.69 28.66,179.01
S$4153
  Bottom 0: 28.66,179.01 28.52,179.31
S$4154
  Bottom 0: 28.52,179.31 28.31,179.55
S$4155
  Bottom 0: 28.31,179.55 28.03,179.73
S$4156
  Bottom 0: 28.03,179.73 27.72,179.82
S$4157
  Bottom 0: 27.72,179.82 27.4,179.82
S$4158
  Bottom 0: 27.4,179.82 27.08,179.73
S$4159
  Bottom 0: 27.08,179.73 26.81,179.55
S$4160
  Bottom 0: 26.81,179.55 26.6,179.31
S$4161
  Bottom 0: 26.6,179.31 26.46,179.01
S$4162
  Bottom 0: 26.46,179.01 26.42,178.69
S$4163
  Bottom 0: 26.42,178.69 26.46,178.37
S$4164
  Bottom 0: 26.46,178.37 26.6,178.07
S$4165
  Bottom 0: 26.6,178.07 26.81,177.82
S$4166
  Bottom 0: 26.81,177.82 27.08,177.65
S$4167
  Bottom 0: 27.08,177.65 27.4,177.56
S$4168
  Bottom 0: 282.82,178.95 283.51,178.95
S$4169
  Bottom 0: 283.51,178.95 283.47,179.06
S$4170
  Bottom 0: 283.47,179.06 283.27,179.34
S$4171
  Bottom 0: 283.27,179.34 283,179.56
S$4172
  Bottom 0: 283,179.56 282.82,179.64
S$4173
  Bottom 0: 282.82,179.64 282.82,178.95
S$4174
  Bottom 0: 280.97,178.95 281.67,178.95
S$4175
  Bottom 0: 281.67,178.95 281.67,179.66
S$4176
  Bottom 0: 281.67,179.66 281.64,179.65
S$4177
  Bottom 0: 281.64,179.65 281.35,179.46
S$4178
  Bottom 0: 281.35,179.46 281.11,179.2
S$4179
  Bottom 0: 281.11,179.2 280.97,178.95
S$4180
  Bottom 0: 18.1,91.84 18.11,91.85
S$4181
  Bottom 0: 18.11,91.85 18.32,92.06
S$4182
  Bottom 0: 18.32,92.06 18.39,92.2
S$4183
  Bottom 0: 18.39,92.2 22.2,92.2
S$4184
  Bottom 0: 22.2,92.2 22.27,92.2
S$4185
  Bottom 0: 22.27,92.2 22.34,92.22
S$4186
  Bottom 0: 22.34,92.22 22.4,92.24
S$4187
  Bottom 0: 22.4,92.24 22.46,92.28
S$4188
  Bottom 0: 22.46,92.28 22.51,92.32
S$4189
  Bottom 0: 22.51,92.32 29.65,99.46
S$4190
  Bottom 0: 29.65,99.46 32.45,99.46
S$4191
  Bottom 0: 32.45,99.46 32.16,99.31
S$4192
  Bottom 0: 32.16,99.31 31.82,99.02
S$4193
  Bottom 0: 31.82,99.02 31.53,98.68
S$4194
  Bottom 0: 31.53,98.68 31.32,98.28
S$4195
  Bottom 0: 31.32,98.28 31.19,97.86
S$4196
  Bottom 0: 31.19,97.86 31.14,97.41
S$4197
  Bottom 0: 31.14,97.41 31.19,96.96
S$4198
  Bottom 0: 31.19,96.96 31.32,96.53
S$4199
  Bottom 0: 31.32,96.53 31.53,96.14
S$4200
  Bottom 0: 31.53,96.14 31.82,95.79
S$4201
  Bottom 0: 31.82,95.79 32.16,95.51
S$4202
  Bottom 0: 32.16,95.51 32.53,95.31
S$4203
  Bottom 0: 32.53,95.31 25.73,95.31
S$4204
  Bottom 0: 25.73,95.31 25.66,95.31
S$4205
  Bottom 0: 25.66,95.31 25.59,95.29
S$4206
  Bottom 0: 25.59,95.29 25.53,95.27
S$4207
  Bottom 0: 25.53,95.27 25.47,95.22
S$4208
  Bottom 0: 25.47,95.22 25.41,95.18
S$4209
  Bottom 0: 25.41,95.18 22.07,91.84
S$4210
  Bottom 0: 22.07,91.84 18.1,91.84
S$4211
  Bottom 0: 18.39,93.08 18.32,93.21
S$4212
  Bottom 0: 18.32,93.21 18.11,93.43
S$4213
  Bottom 0: 18.11,93.43 17.85,93.58
S$4214
  Bottom 0: 17.85,93.58 17.56,93.65
S$4215
  Bottom 0: 17.56,93.65 17.25,93.63
S$4216
  Bottom 0: 17.25,93.63 16.97,93.52
S$4217
  Bottom 0: 16.97,93.52 16.73,93.33
S$4218
  Bottom 0: 16.73,93.33 16.61,93.14
S$4219
  Bottom 0: 16.61,93.14 16.61,94.28
S$4220
  Bottom 0: 16.61,94.28 16.6,94.35
S$4221
  Bottom 0: 16.6,94.35 16.59,94.42
S$4222
  Bottom 0: 16.59,94.42 16.56,94.48
S$4223
  Bottom 0: 16.56,94.48 16.52,94.54
S$4224
  Bottom 0: 16.52,94.54 16.48,94.59
S$4225
  Bottom 0: 16.48,94.59 10.05,101.03
S$4226
  Bottom 0: 10.05,101.03 10.05,101.74
S$4227
  Bottom 0: 10.05,101.74 10.14,101.62
S$4228
  Bottom 0: 10.14,101.62 10.42,101.45
S$4229
  Bottom 0: 10.42,101.45 10.73,101.36
S$4230
  Bottom 0: 10.73,101.36 11.05,101.36
S$4231
  Bottom 0: 11.05,101.36 11.36,101.45
S$4232
  Bottom 0: 11.36,101.45 11.64,101.62
S$4233
  Bottom 0: 11.64,101.62 11.85,101.87
S$4234
  Bottom 0: 11.85,101.87 11.87,101.92
S$4235
  Bottom 0: 11.87,101.92 13.87,101.92
S$4236
  Bottom 0: 13.87,101.92 13.96,101.92
S$4237
  Bottom 0: 13.96,101.92 14.05,101.94
S$4238
  Bottom 0: 14.05,101.94 14.13,101.98
S$4239
  Bottom 0: 14.13,101.98 14.2,102.03
S$4240
  Bottom 0: 14.2,102.03 14.27,102.09
S$4241
  Bottom 0: 14.27,102.09 26.66,114.49
S$4242
  Bottom 0: 26.66,114.49 34.13,107.02
S$4243
  Bottom 0: 34.13,107.02 34.13,103.47
S$4244
  Bottom 0: 34.13,103.47 33.95,103.35
S$4245
  Bottom 0: 33.95,103.35 33.74,103.11
S$4246
  Bottom 0: 33.74,103.11 33.6,102.81
S$4247
  Bottom 0: 33.6,102.81 33.56,102.49
S$4248
  Bottom 0: 33.56,102.49 33.6,102.17
S$4249
  Bottom 0: 33.6,102.17 33.74,101.87
S$4250
  Bottom 0: 33.74,101.87 33.95,101.62
S$4251
  Bottom 0: 33.95,101.62 34.23,101.45
S$4252
  Bottom 0: 34.23,101.45 34.54,101.36
S$4253
  Bottom 0: 34.54,101.36 34.86,101.36
S$4254
  Bottom 0: 34.86,101.36 34.91,101.37
S$4255
  Bottom 0: 34.91,101.37 33.89,100.34
S$4256
  Bottom 0: 33.89,100.34 29.46,100.34
S$4257
  Bottom 0: 29.46,100.34 29.39,100.34
S$4258
  Bottom 0: 29.39,100.34 29.32,100.33
S$4259
  Bottom 0: 29.32,100.33 29.27,100.3
S$4260
  Bottom 0: 29.27,100.3 29.2,100.26
S$4261
  Bottom 0: 29.2,100.26 29.15,100.22
S$4262
  Bottom 0: 29.15,100.22 22.01,93.08
S$4263
  Bottom 0: 22.01,93.08 18.39,93.08
S$4264
  Bottom 0: 21.27,95.89 21.79,95.89
S$4265
  Bottom 0: 21.79,95.89 22.29,95.98
S$4266
  Bottom 0: 22.29,95.98 22.79,96.14
S$4267
  Bottom 0: 22.79,96.14 23.24,96.39
S$4268
  Bottom 0: 23.24,96.39 23.65,96.71
S$4269
  Bottom 0: 23.65,96.71 24,97.09
S$4270
  Bottom 0: 24,97.09 24.29,97.52
S$4271
  Bottom 0: 24.29,97.52 24.5,98
S$4272
  Bottom 0: 24.5,98 24.62,98.5
S$4273
  Bottom 0: 24.62,98.5 24.66,99.01
S$4274
  Bottom 0: 24.66,99.01 24.62,99.53
S$4275
  Bottom 0: 24.62,99.53 24.5,100.03
S$4276
  Bottom 0: 24.5,100.03 24.29,100.51
S$4277
  Bottom 0: 24.29,100.51 24,100.94
S$4278
  Bottom 0: 24,100.94 23.65,101.32
S$4279
  Bottom 0: 23.65,101.32 23.24,101.64
S$4280
  Bottom 0: 23.24,101.64 22.79,101.88
S$4281
  Bottom 0: 22.79,101.88 22.29,102.05
S$4282
  Bottom 0: 22.29,102.05 21.79,102.14
S$4283
  Bottom 0: 21.79,102.14 21.27,102.14
S$4284
  Bottom 0: 21.27,102.14 20.76,102.05
S$4285
  Bottom 0: 20.76,102.05 20.27,101.88
S$4286
  Bottom 0: 20.27,101.88 19.82,101.64
S$4287
  Bottom 0: 19.82,101.64 19.4,101.32
S$4288
  Bottom 0: 19.4,101.32 19.05,100.94
S$4289
  Bottom 0: 19.05,100.94 18.77,100.51
S$4290
  Bottom 0: 18.77,100.51 18.56,100.03
S$4291
  Bottom 0: 18.56,100.03 18.43,99.53
S$4292
  Bottom 0: 18.43,99.53 18.39,99.01
S$4293
  Bottom 0: 18.39,99.01 18.43,98.5
S$4294
  Bottom 0: 18.43,98.5 18.56,98
S$4295
  Bottom 0: 18.56,98 18.77,97.52
S$4296
  Bottom 0: 18.77,97.52 19.05,97.09
S$4297
  Bottom 0: 19.05,97.09 19.4,96.71
S$4298
  Bottom 0: 19.4,96.71 19.82,96.39
S$4299
  Bottom 0: 19.82,96.39 20.27,96.14
S$4300
  Bottom 0: 20.27,96.14 20.76,95.98
S$4301
  Bottom 0: 20.76,95.98 21.27,95.89
S$4302
  Bottom 0: 31.27,101.35 33.05,101.35
S$4303
  Bottom 0: 33.05,101.35 33.13,101.36
S$4304
  Bottom 0: 33.13,101.36 33.2,101.4
S$4305
  Bottom 0: 33.2,101.4 33.25,101.45
S$4306
  Bottom 0: 33.25,101.45 33.29,101.52
S$4307
  Bottom 0: 33.29,101.52 33.3,101.6
S$4308
  Bottom 0: 33.3,101.6 33.3,103.38
S$4309
  Bottom 0: 33.3,103.38 33.29,103.45
S$4310
  Bottom 0: 33.29,103.45 33.25,103.53
S$4311
  Bottom 0: 33.25,103.53 33.2,103.58
S$4312
  Bottom 0: 33.2,103.58 33.13,103.62
S$4313
  Bottom 0: 33.13,103.62 33.05,103.63
S$4314
  Bottom 0: 33.05,103.63 31.27,103.63
S$4315
  Bottom 0: 31.27,103.63 31.2,103.62
S$4316
  Bottom 0: 31.2,103.62 31.12,103.58
S$4317
  Bottom 0: 31.12,103.58 31.07,103.53
S$4318
  Bottom 0: 31.07,103.53 31.03,103.45
S$4319
  Bottom 0: 31.03,103.45 31.02,103.38
S$4320
  Bottom 0: 31.02,103.38 31.02,101.6
S$4321
  Bottom 0: 31.02,101.6 31.03,101.52
S$4322
  Bottom 0: 31.03,101.52 31.07,101.45
S$4323
  Bottom 0: 31.07,101.45 31.12,101.4
S$4324
  Bottom 0: 31.12,101.4 31.2,101.36
S$4325
  Bottom 0: 31.2,101.36 31.27,101.35
S$4326
  Bottom 0: 206.31,93.12 205.18,94.25
S$4327
  Bottom 0: 205.18,94.25 205.28,94.52
S$4328
  Bottom 0: 205.28,94.52 205.33,94.87
S$4329
  Bottom 0: 205.33,94.87 205.28,95.21
S$4330
  Bottom 0: 205.28,95.21 205.16,95.54
S$4331
  Bottom 0: 205.16,95.54 204.95,95.82
S$4332
  Bottom 0: 204.95,95.82 204.68,96.05
S$4333
  Bottom 0: 204.68,96.05 204.37,96.19
S$4334
  Bottom 0: 204.37,96.19 204.37,101.8
S$4335
  Bottom 0: 204.37,101.8 204.37,101.87
S$4336
  Bottom 0: 204.37,101.87 204.35,101.94
S$4337
  Bottom 0: 204.35,101.94 204.33,102.01
S$4338
  Bottom 0: 204.33,102.01 204.29,102.06
S$4339
  Bottom 0: 204.29,102.06 204.24,102.12
S$4340
  Bottom 0: 204.24,102.12 196.73,109.62
S$4341
  Bottom 0: 196.73,109.62 196.68,109.66
S$4342
  Bottom 0: 196.68,109.66 196.62,109.7
S$4343
  Bottom 0: 196.62,109.7 196.56,109.73
S$4344
  Bottom 0: 196.56,109.73 196.49,109.74
S$4345
  Bottom 0: 196.49,109.74 196.42,109.75
S$4346
  Bottom 0: 196.42,109.75 192.06,109.75
S$4347
  Bottom 0: 192.06,109.75 188.5,113.3
S$4348
  Bottom 0: 188.5,113.3 188.61,113.57
S$4349
  Bottom 0: 188.61,113.57 188.66,113.92
S$4350
  Bottom 0: 188.66,113.92 188.61,114.26
S$4351
  Bottom 0: 188.61,114.26 188.48,114.59
S$4352
  Bottom 0: 188.48,114.59 188.28,114.87
S$4353
  Bottom 0: 188.28,114.87 188.01,115.1
S$4354
  Bottom 0: 188.01,115.1 187.69,115.25
S$4355
  Bottom 0: 187.69,115.25 187.34,115.31
S$4356
  Bottom 0: 187.34,115.31 187,115.29
S$4357
  Bottom 0: 187,115.29 186.99,115.29
S$4358
  Bottom 0: 186.99,115.29 191.76,120.06
S$4359
  Bottom 0: 191.76,120.06 192.07,120.06
S$4360
  Bottom 0: 192.07,120.06 192.24,119.81
S$4361
  Bottom 0: 192.24,119.81 192.48,119.62
S$4362
  Bottom 0: 192.48,119.62 192.76,119.51
S$4363
  Bottom 0: 192.76,119.51 193.06,119.49
S$4364
  Bottom 0: 193.06,119.49 193.36,119.56
S$4365
  Bottom 0: 193.36,119.56 193.62,119.71
S$4366
  Bottom 0: 193.62,119.71 193.82,119.93
S$4367
  Bottom 0: 193.82,119.93 193.96,120.2
S$4368
  Bottom 0: 193.96,120.2 194,120.5
S$4369
  Bottom 0: 194,120.5 193.96,120.8
S$4370
  Bottom 0: 193.96,120.8 193.82,121.08
S$4371
  Bottom 0: 193.82,121.08 193.62,121.3
S$4372
  Bottom 0: 193.62,121.3 193.36,121.45
S$4373
  Bottom 0: 193.36,121.45 193.06,121.51
S$4374
  Bottom 0: 193.06,121.51 192.89,121.5
S$4375
  Bottom 0: 192.89,121.5 197.05,125.67
S$4376
  Bottom 0: 197.05,125.67 197.92,125.67
S$4377
  Bottom 0: 197.92,125.67 197.78,125.54
S$4378
  Bottom 0: 197.78,125.54 197.61,125.27
S$4379
  Bottom 0: 197.61,125.27 197.53,124.95
S$4380
  Bottom 0: 197.53,124.95 197.53,124.63
S$4381
  Bottom 0: 197.53,124.63 197.61,124.31
S$4382
  Bottom 0: 197.61,124.31 197.78,124.04
S$4383
  Bottom 0: 197.78,124.04 198.02,123.81
S$4384
  Bottom 0: 198.02,123.81 198.31,123.67
S$4385
  Bottom 0: 198.31,123.67 198.63,123.6
S$4386
  Bottom 0: 198.63,123.6 198.95,123.62
S$4387
  Bottom 0: 198.95,123.62 199.18,123.7
S$4388
  Bottom 0: 199.18,123.7 200.23,122.65
S$4389
  Bottom 0: 200.23,122.65 200.19,122.63
S$4390
  Bottom 0: 200.19,122.63 200.14,122.58
S$4391
  Bottom 0: 200.14,122.58 200.1,122.5
S$4392
  Bottom 0: 200.1,122.5 200.09,122.43
S$4393
  Bottom 0: 200.09,122.43 200.09,120.65
S$4394
  Bottom 0: 200.09,120.65 200.1,120.57
S$4395
  Bottom 0: 200.1,120.57 200.14,120.5
S$4396
  Bottom 0: 200.14,120.5 200.19,120.45
S$4397
  Bottom 0: 200.19,120.45 200.26,120.41
S$4398
  Bottom 0: 200.26,120.41 200.34,120.4
S$4399
  Bottom 0: 200.34,120.4 202.12,120.4
S$4400
  Bottom 0: 202.12,120.4 202.19,120.41
S$4401
  Bottom 0: 202.19,120.41 202.26,120.45
S$4402
  Bottom 0: 202.26,120.45 202.32,120.5
S$4403
  Bottom 0: 202.32,120.5 202.36,120.57
S$4404
  Bottom 0: 202.36,120.57 202.37,120.65
S$4405
  Bottom 0: 202.37,120.65 202.37,122.43
S$4406
  Bottom 0: 202.37,122.43 202.36,122.49
S$4407
  Bottom 0: 202.36,122.49 202.77,122.08
S$4408
  Bottom 0: 202.77,122.08 202.67,121.86
S$4409
  Bottom 0: 202.67,121.86 202.63,121.54
S$4410
  Bottom 0: 202.63,121.54 202.67,121.22
S$4411
  Bottom 0: 202.67,121.22 202.81,120.92
S$4412
  Bottom 0: 202.81,120.92 203.02,120.67
S$4413
  Bottom 0: 203.02,120.67 203.3,120.5
S$4414
  Bottom 0: 203.3,120.5 203.6,120.41
S$4415
  Bottom 0: 203.6,120.41 203.93,120.41
S$4416
  Bottom 0: 203.93,120.41 204.24,120.5
S$4417
  Bottom 0: 204.24,120.5 204.52,120.67
S$4418
  Bottom 0: 204.52,120.67 204.73,120.92
S$4419
  Bottom 0: 204.73,120.92 204.87,121.22
S$4420
  Bottom 0: 204.87,121.22 204.91,121.54
S$4421
  Bottom 0: 204.91,121.54 204.87,121.86
S$4422
  Bottom 0: 204.87,121.86 204.73,122.16
S$4423
  Bottom 0: 204.73,122.16 204.52,122.4
S$4424
  Bottom 0: 204.52,122.4 204.24,122.58
S$4425
  Bottom 0: 204.24,122.58 203.93,122.67
S$4426
  Bottom 0: 203.93,122.67 203.78,122.67
S$4427
  Bottom 0: 203.78,122.67 199.82,126.64
S$4428
  Bottom 0: 199.82,126.64 199.75,126.7
S$4429
  Bottom 0: 199.75,126.7 199.67,126.75
S$4430
  Bottom 0: 199.67,126.75 199.59,126.78
S$4431
  Bottom 0: 199.59,126.78 199.51,126.8
S$4432
  Bottom 0: 199.51,126.8 199.41,126.81
S$4433
  Bottom 0: 199.41,126.81 199.2,126.81
S$4434
  Bottom 0: 199.2,126.81 199.2,136.21
S$4435
  Bottom 0: 199.2,136.21 199.19,136.3
S$4436
  Bottom 0: 199.19,136.3 199.17,136.38
S$4437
